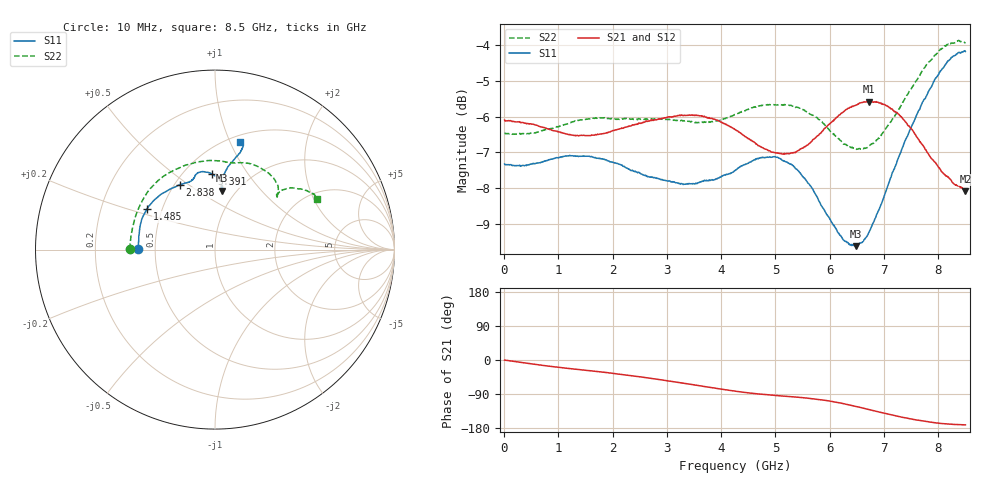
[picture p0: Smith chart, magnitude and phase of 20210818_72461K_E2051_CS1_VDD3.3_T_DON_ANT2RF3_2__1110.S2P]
!Agilent Technologies,E5071C,MY46417908,A.11.23
!Date: Wed Aug 18 14:30:08 2021
!Data & Calibration Information:
!Freq	S11:SOLT2(ON)	S21:SOLT2(ON)	S12:SOLT2(ON)	S22:SOLT2(ON)
!PortZ  Port1:50+j0  Port2:50+j0
!Above PortZ is port z conversion or system Z0 setting when saving the data.
!When reading, reference impedance value at option line is always used.
# Hz S dB R 50
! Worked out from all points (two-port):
!   1601 points, 10 MHz to 8.5 GHz, reference 50 ohm
!   highest |S21| = -5.58 dB at 6.722 GHz (marker M1); lowest = -8.1 dB at 8.5 GHz (marker M2)
!   |S21| within 3 dB of the highest: start of sweep to end of sweep
!   lowest |S11| = -9.6 dB at 6.489 GHz (marker M3), VSWR 1.99, Z = 43 + j31.7 ohm
!   |S11| at or under -10 dB: nowhere
!   |S22| runs from -6.9 to -3.9 dB; largest |S21 - S12| = 0.0032
!   S11 on the Smith chart (normalised r, x): 10 MHz: 0.40, +0.00; 1.485 GHz: 0.41, +0.23; 2.838 GHz: 0.53, +0.46; 5.391 GHz: 0.68, +0.70; 8.5 GHz: 0.56, +1.09
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1e7  -7.32 179.7  -6.10 -0.4  -6.10 -0.3  -6.45 179.6
7.847125e8  -7.23 164.8  -6.33 -15.5  -6.33 -15.5  -6.36 156.5
1.426769e9  -7.11 150.7  -6.52 -26.0  -6.53 -25.9  -6.09 135.6
1.485138e9  -7.11 149.2  -6.53 -26.9  -6.54 -26.9  -6.09 133.6
1.803512e9  -7.18 141.6  -6.48 -31.8  -6.49 -31.8  -6.04 123.5
2.206788e9  -7.39 132.1  -6.31 -38.7  -6.31 -38.7  -6.06 111.0
2.838231e9  -7.73 118.3  -6.08 -51.2  -6.08 -51.2  -6.07 94.7
2.843538e9  -7.74 118.3  -6.07 -51.3  -6.07 -51.3  -6.07 94.7
3.61825e9  -7.82 108.7  -5.98 -68.4  -5.97 -68.4  -6.16 81.7
4.255e9  -7.51 105.5  -6.36 -82.1  -6.35 -82.2  -5.94 73.7
4.801544e9  -7.15 101.6  -6.91 -91.1  -6.90 -91.1  -5.69 64.7
5.390538e9  -7.47 92.5  -6.98 -98.0  -6.98 -98.0  -5.74 51.8
5.671769e9  -8.00 87.8  -6.69 -101.9  -6.71 -101.9  -5.96 46.7
5.921162e9  -8.67 84.3  -6.31 -106.6  -6.34 -106.6  -6.26 43.6
6.159944e9  -9.25 83.1  -5.98 -112.5  -6.00 -112.6  -6.62 41.4
6.488931e9  -9.62 83.6  -5.69 -122.7  -5.68 -122.8  -6.92 40.5
6.722406e9  -9.24 84.1  -5.58 -130.7  -5.58 -130.9  -6.83 41.1
7.088538e9  -7.85 83.5  -5.74 -143.3  -5.74 -143.3  -6.22 41.7
7.385688e9  -6.69 81.3  -6.13 -152.5  -6.13 -152.7  -5.50 40.1
7.836719e9  -5.26 76.2  -7.09 -163.6  -7.06 -163.8  -4.47 34.1
8.165706e9  -4.47 74.9  -7.68 -168.7  -7.65 -168.8  -4.00 29.4
8.5e9  -4.18 77.1  -8.09 -171.2  -8.03 -171.2  -3.96 26.5
